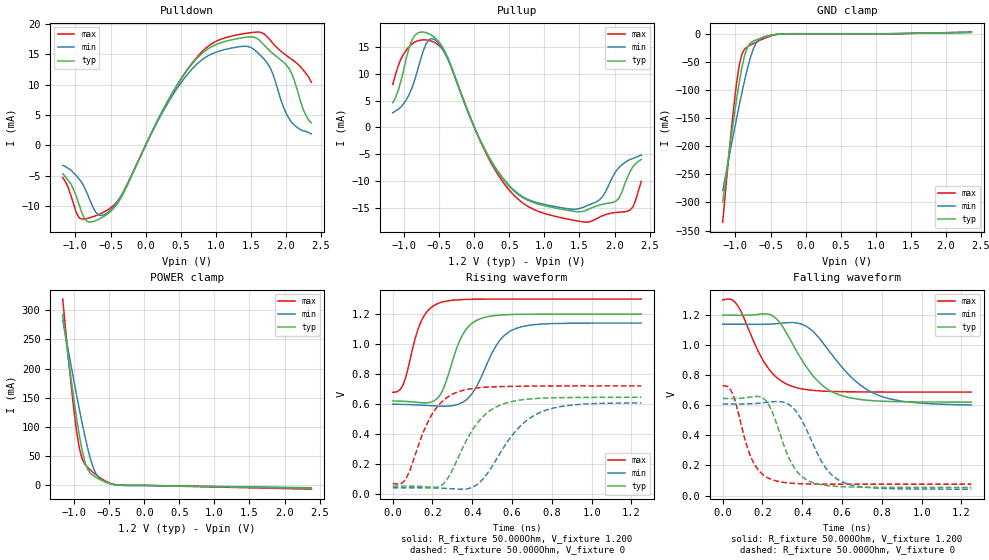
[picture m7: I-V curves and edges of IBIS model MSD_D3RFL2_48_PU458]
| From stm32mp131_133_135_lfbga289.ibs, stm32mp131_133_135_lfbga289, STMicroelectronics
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[Model] MSD_D3RFL2_48_PU458
Model_type   I/O
C_comp 2.406pF   2.319pF   2.532pF
Vinh = 820.000mV
Vinl = 380.000mV
Vmeas = 600.000mV
Vref = 600.000mV
[Model Spec]
Vinh   820.000mV   790.000mV   870.000mV
Vinl   380.000mV   350.000mV   430.000mV
Vmeas   600.000mV   570.000mV   650.000mV
Vref   600.000mV   570.000mV   650.000mV
[Receiver Thresholds]
Vth   =  0.600V
Vth_min  =  0.5880V
Vth_max  =  0.6120V
Vinh_ac  =  0.220V
Vinh_dc  =  0.130V
Vinl_ac  = -0.220V
Vinl_dc  = -0.130V
Tslew_ac =  5.000ns |Not specified, so set to high value
[Temperature Range]   25.000   125.000   -40.000
[Voltage Range]   1.200V   1.140V   1.300V
[GND Clamp Reference]   0.00V   0.00V   0.00V
[Pulldown Reference]   0.00V   0.00V   0.00V
[POWER Clamp Reference]   1.200V   1.140V   1.300V
[Pullup Reference]   1.200V   1.140V   1.300V
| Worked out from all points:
|   slope of the pulldown table from 0 to 0.18 V, typ, clamps not added: 41.6 ohm
|   slope of the pullup table from 0 to 0.18 V, typ, clamps not added: 36.3 ohm
|   GND clamp passes 1 mA (typ) near -0.40 V on its own axis
|   POWER clamp passes 1 mA (typ) near -0.41 V on its own axis
|   rising waveform, R_fixture 50.000Ohm, V_fixture 1.200: 20-80 % time 97.3ps typ, 126ps min, 82.2ps max; typ from 0.621 V to 1.2 V
|   rising waveform, R_fixture 50.000Ohm, V_fixture 0: 20-80 % time 158ps typ, 192ps min, 132ps max; typ from 0.054 V to 0.646 V
|   falling waveform, R_fixture 50.000Ohm, V_fixture 1.200: 20-80 % time 177ps typ, 225ps min, 144ps max; typ from 1.2 V to 0.622 V
|   falling waveform, R_fixture 50.000Ohm, V_fixture 0: 20-80 % time 109ps typ, 135ps min, 92.1ps max; typ from 0.646 V to 0.054 V
[GND Clamp]
-1.182V   -299mA     -279mA     -335.2mA
-1.064V   -186.9mA   -201.3mA   -176.9mA
-984.9mV  -117.5mA   -151.2mA   -88.11mA
-945.5mV  -86.15mA   -126.9mA   -55.31mA
-906.1mV  -58.77mA   -103.6mA   -35.22mA
-866.7mV  -37.28mA   -81.4mA    -26.82mA
-827.3mV  -23.51mA   -60.86mA   -23.06mA
-748.5mV  -13.37mA   -27.9mA    -17.67mA
-709.1mV  -11.21mA   -17.31mA   -15.18mA
-630.3mV  -7.712mA   -7.374mA   -10.51mA
-472.7mV  -2.381mA   -2.076mA   -3.096mA
2.364V    2.48mA     2.095mA    2.917mA
[Power Clamp]
-1.164V   292.1mA    282.5mA    318.8mA
-1.085V   218.4mA    230.8mA    219.7mA
-1.006V   148.3mA    180mA      130.8mA
-966.7mV  115.6mA    155.1mA    93.04mA
-927.3mV  85.92mA    130.8mA    63.68mA
-887.9mV  60.21mA    107.3mA    45.58mA
-809.1mV  27.67mA    64.23mA    30.9mA
-730.3mV  16.91mA    31.08mA    22.23mA
-690.9mV  13.83mA    20.26mA    18.38mA
-572.7mV  6.582mA    6.523mA    8.677mA
-336.4mV  195.4uA    370.9uA    217.1uA
2.382V    -4.955mA   -3.949mA   -6.434mA
[Pulldown]
-1.182V   -4.7mA     -3.3mA     -5.3mA
-945.5mV  -9.88mA    -5.6mA     -11.97mA
-827.3mV  -12.62mA   -8.09mA    -12.05mA
-709.1mV  -12.41mA   -11.06mA   -11.6mA
-551.5mV  -11.39mA   -11.19mA   -10.72mA
-315.1mV  -7.913mA   -7.696mA   -7.646mA
551.5mV   11.71mA    11.03mA    11.75mA
906.1mV   16.03mA    14.86mA    16.45mA
1.261V    17.48mA    16.11mA    18.1mA
1.733V    16.03mA    13.62mA    17.93mA
2.009V    13.23mA    5.15mA     14.8mA
2.364V    3.7mA      1.9mA      10.4mA
[Pullup]
-1.164V   4.6mA      2.709mA    7.977mA
-1.045V   8.7mA      3.814mA    12.81mA
-887.9mV  16.31mA    7.406mA    15.56mA
-612.1mV  17.19mA    16.55mA    16.09mA
-375.8mV  12.93mA    12.63mA    12.73mA
215.2mV   -5.799mA   -5.653mA   -6.081mA
687.9mV   -13.07mA   -12.91mA   -14.07mA
1.476V    -15.75mA   -15.22mA   -17.47mA
1.791V    -14.48mA   -13.46mA   -16.71mA
1.988V    -13.96mA   -8.894mA   -15.94mA
2.224V    -8.2mA     -5.995mA   -15.42mA
2.382V    -6mA       -5.195mA   -10.06mA
[Ramp]
R_load=50.000Ohm
dV/dt_r   351.399mV/128.500ps  332.358mV/161.000ps  377.424mV/106.500ps
dV/dt_f   351.369mV/144.000ps  332.355mV/182.000ps  377.424mV/118.500ps
[Rising waveform]
R_fixture=50.000Ohm
V_fixture=1.200
V_fixture_min=1.140
V_fixture_max=1.300
0s        621.1mV    599.4mV    679mV
52ps      619mV      598.1mV    728.5mV
115ps     612.8mV    594.9mV    1.047V
154ps     608.8mV    592.2mV    1.18V
230ps     645.8mV    586.8mV    1.272V
345ps     1.046V     607.9mV    1.296V
435ps     1.166V     752.3mV    1.299V
537ps     1.193V     1.022V     1.3V
626ps     1.198V     1.107V     1.3V
1.25ns    1.2V       1.14V      1.3V
[Rising waveform]
R_fixture=50.000Ohm
V_fixture=0
0s        53.83mV    42.15mV    71.37mV
64ps      54.22mV    42.43mV    98.19mV
166ps     49.08mV    42.36mV    450.2mV
230ps     48.86mV    40.78mV    592mV
320ps     216.5mV    34.41mV    677.6mV
435ps     489.4mV    75.62mV    709.4mV
549ps     598.1mV    293.4mV    717.1mV
652ps     629.2mV    467.1mV    719.3mV
779ps     641.2mV    563.6mV    720.6mV
1.25ns    645.6mV    608.2mV    721.2mV
[Falling waveform]
R_fixture=50.000Ohm
V_fixture=1.200
V_fixture_min=1.140
V_fixture_max=1.300
0s        1.2V       1.14V      1.302V
77ps      1.199V     1.14V      1.26V
179ps     1.205V     1.139V     958.5mV
243ps     1.201V     1.141V     823.3mV
345ps     1.024V     1.151V     728.1mV
460ps     785.6mV    1.084V     698.6mV
600ps     663.7mV    853.1mV    690.8mV
715ps     635.5mV    713.6mV    689mV
830ps     626mV      646.1mV    688.5mV
1.25ns    621.5mV    602.5mV    688.2mV
[Falling waveform]
R_fixture=50.000Ohm
V_fixture=0
0s        645.6mV    609.1mV    729.3mV
52ps      645.4mV    608.8mV    670.7mV
154ps     657.8mV    611.3mV    222.1mV
205ps     646.3mV    617.2mV    136.3mV
243ps     574.4mV    622.7mV    108.1mV
345ps     218.4mV    593.2mV    81.88mV
447ps     88.37mV    363.1mV    76.37mV
524ps     66.16mV    172.6mV    75.39mV
626ps     57.3mV     77.67mV    75.07mV
1.25ns    53.68mV    42.16mV    74.93mV
